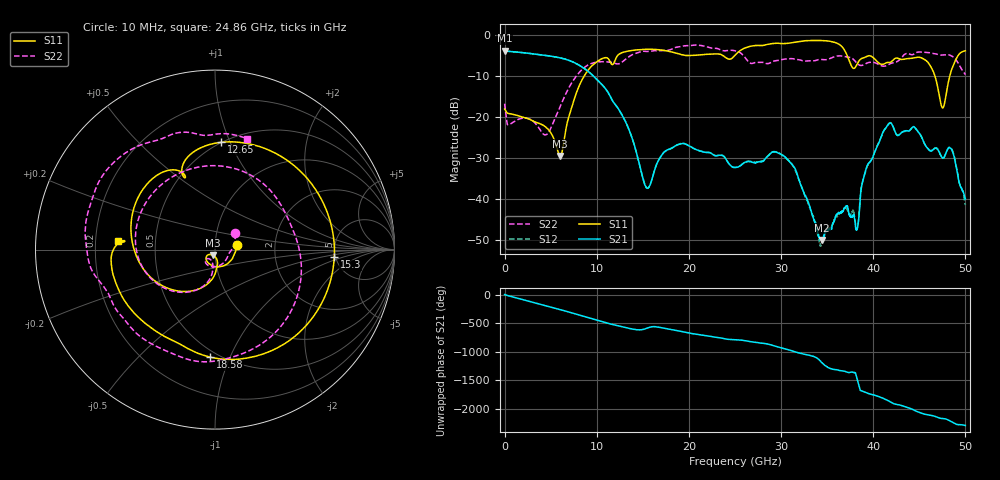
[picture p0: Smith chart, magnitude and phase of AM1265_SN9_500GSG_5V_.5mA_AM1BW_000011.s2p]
!Keysight Technologies,N5245B,MY58422270,A.16.20.02
!Date: Thursday, March 05, 2026 00:27:34
!Correction: S11(C  2-Port  )
!S21(C  2-Port  )
!S12(C  2-Port  )
!S22(C  2-Port  )
!S2P File: Measurements: S11, S21, S12, S22:
# Hz S  dB  R 50
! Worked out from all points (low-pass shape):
!   3201 points, 10 MHz to 50 GHz, reference 50 ohm
!   highest |S21| = -3.86 dB at 10 MHz (marker M1); lowest = -50.0 dB at 34.46 GHz (marker M2)
!   |S21| within 3 dB of the highest: start of sweep to 7.641 GHz
!   lowest |S11| = -29.6 dB at 6.04 GHz (marker M3), VSWR 1.07, Z = 48.6 - j2.95 ohm
!   |S11| at or under -10 dB: start of sweep to 8.657 GHz; 46.69 GHz to 48.31 GHz (1.621 GHz wide, 3.41 % of centre)
!   |S22| runs from -24.4 to -2.5 dB; largest |S21 - S12| = 0.01
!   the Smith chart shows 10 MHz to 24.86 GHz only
!   S11 on the Smith chart (normalised r, x): 10 MHz: 1.28, +0.07; 12.65 GHz: 0.50, +0.93; 15.3 GHz: 4.87, -0.74; 18.58 GHz: 0.45, -0.85; 24.86 GHz: 0.30, +0.04
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1e7  -18.10 12.1  -3.86 3.2  -3.81 2.4  -16.80 38.5
2.322038e9  -20.28 -83.1  -4.43 -98.6  -4.44 -98.6  -20.30 -108.1
4.165419e9  -22.01 -124.8  -4.92 -177.1  -4.92 -177.1  -24.09 -126.8
6.040044e9  -29.56 -114.3  -5.62 99.7  -5.63 99.8  -17.47 -97.0
8.352081e9  -11.23 -122.1  -7.77 -9.1  -7.76 -9.0  -8.59 -148.6
1.102342e10  -5.57 130.8  -13.34 -132.5  -13.35 -132.6  -6.58 99.3
1.26481e10  -4.45 86.6  -19.14 163.6  -19.13 163.6  -6.81 7.9
1.530382e10  -3.53 -3.6  -36.99 124.8  -36.90 124.8  -4.06 -109.0
1.667854e10  -3.63 -44.5  -30.71 152.4  -30.64 152.9  -3.92 -141.4
1.858441e10  -4.44 -92.5  -27.00 97.2  -27.03 97.2  -3.06 -172.9
2.48644e10  -5.33 175.1  -32.32 -66.1  -32.31 -66.2  -3.83 74.1
2.5005e10  -4.99 174.1  -32.36 -66.9  -32.33 -67.2  -3.89 70.8
2.947286e10  -2.07 96.6  -28.59 174.3  -28.53 174.8  -6.29 -18.6
3.334708e10  -1.40 35.6  -43.69 6.1  -43.25 6.7  -6.36 -127.7
3.445623e10  -1.41 16.2  -49.97 -114.3  -50.70 -49.9  -6.01 -151.2
3.675265e10  -3.29 -32.8  -42.83 104.6  -42.67 100.2  -5.23 164.2
3.823673e10  -7.22 -22.0  -47.34 -22.8  -47.29 -108.0  -6.96 137.4
3.918966e10  -5.39 -33.1  -32.94 89.1  -33.29 87.6  -7.04 136.2
4.167354e10  -6.76 -54.2  -21.73 -59.5  -21.69 -59.0  -7.24 116.3
4.509473e10  -5.53 -101.6  -24.27 93.3  -24.26 92.9  -4.17 75.6
4.770358e10  -17.04 69.1  -29.79 -10.7  -29.82 -10.8  -4.89 39.5
5e10  -3.89 -72.6  -40.03 -129.6  -41.49 -142.4  -9.70 3.9
